(* Logix 5000 AddOnInstructionDefinition export NORD_VFDcontrol_PRO_Inst100_101; software revision 24.02 *)

TYPE FI_Data_IN :
STRUCT
   ConnectionFaulted : BOOL;
   RunMode : BOOL;
   Data : INT[6];   // Actual Values
END_STRUCT
END_TYPE

TYPE FI_Data_OUT :
STRUCT
   Data : INT[6];   // Control Data
END_STRUCT
END_TYPE

ADD_ON_INSTRUCTION NORD_VFDcontrol_PRO_Inst100_101   (* revision 1.1, vendor NORD Drivesystems, ExecutePrescan *)
// Control Block for NORD SK 5xxP VFD
// Revision note:
// Rev 1.1
// Better Ready Start Condition Logic
// Added Inhibited Output
// Added Fault Active Output
// Rev 1.0
// Connection to SK550P
// Instances: Output 100/Input 101
// For VFD Series:
//    - PRO (SK 500P Series)
// Allows for control of up to four (8) VFDs.
//    - FI_Control/Status may require Data Type change
VAR_IN_OUT
   FI_Status : _0342:XU5_EIP_DE5BFA94:I:0; {required}   // Input Data Map of VFD
   FI_Control : _0342:XU5_EIP_E8E6FFA2:O:0; {required}   // Output Data Map of VFD
END_VAR
VAR_INPUT
   Max_VFD_Number : SINT := 1;   // Maximum Number of VFDs on this specific node (1-8 for Instance 100/101)
   VFD_Number : SINT := 1; {visible}   // Number of VFD to control (1...Max_VFD_Number) for Instance 102/103)
   EnableFwd : BOOL; {visible}   // HIGH = Enable CW
   EnableRev : BOOL; {visible}   // HIGH = Enable CCW
   DisableVoltage : BOOL := 1; {visible}   // LOW = Output Voltage Disabled
   QuickStop : BOOL := 1; {visible}   // LOW = Emergency Stop Active
   FaultAckn : BOOL; {visible}   // Error / Fault Acknowledgement on Rising Edge
   ParameterSet : SINT := 1; {visible}   // Parameter Set 1-4, If less than 1 or higher than 4, Set 1 as active
        .1   // Parameter Set 1-4, If less than 1 or higher than 4, Set 1 as active
   Activate32BitSetpoint : BOOL; {visible}   // Use 32Bit Setpoint
   ControlWordBit8_P480_11 : BOOL; {visible}   // P480_11 - Function
   ControlWordBit9_P480_12 : BOOL; {visible}   // P480_12 - Function
   ControlWord : ALIAS FOR Control_Word; {access None, visible}
   Setpoint1 : INT; {visible}   // Setpoint 1 Function set in P546[1]
   Setpoint2 : INT; {visible}   // Setpoint 2 Function set in P546[2]
   Setpoint3 : INT; {visible}   // Setpoint 3 Function set in P546[3]
   Setpoint2_3_32 : DINT; {visible}   // 32 Bit Setpoint 2
   Setpoint4 : INT; {visible}   // Setpoint 4 Function set in P546[4]
   Setpoint5 : INT; {visible}   // Setpoint 5 Function set in P546[5]
END_VAR
VAR_OUTPUT
   StatusWord : INT; {access Read Only, visible}   // Status Word
        .0   // Ready to Start
        .1   // Ready for Operation
        .2   // Operation Enabled
        .3   // Fault
        .4   // Voltage Enabled
        .5   // No Emergency Stop
        .6   // Starting Disabled
        .7   // Warning Active
        .8   // Setpoint Reached
        .9   // Bus Controller Active
        .10   // Function P481[9]
        .11   // Rotation Right Active
        .12   // Rotation Left Active
        .13   // Function P481[10]
        .14   // Parameter Set Bit 0
        .15   // Parameter Set Bit 1
   ActiveParameterSet : SINT; {access Read Only, visible}   // Displays active parameter set
   CommunicationOK : BOOL; {access Read Only, visible}   // Communication is OK
   ReadyToStart : BOOL; {access Read Only, visible}   // Drive Ready to Start
   VFD_Enabled : BOOL; {access Read Only, visible}   // VFD is Enabled
   Inhibited : BOOL; {access Read Only, visible}   // VFD is Inhibited
   Warning : BOOL; {access Read Only, visible}   // Drive has a Warning
   Faulted : BOOL; {access Read Only, visible}   // Drive Faulted
   FaultActive : BOOL; {access Read Only, visible}   // Fault Conditions are Currently Active
   StatusWordBit10_P481_9 : BOOL; {access Read Only, visible}   // P481_09 - Function
   StatusWordBit13_P481_10 : BOOL; {access Read Only, visible}   // P481_10 - Function
   ActualValue1 : INT; {access Read Only, visible}   // Actual Value 1 Function set in P543[1]
   ActualValue2 : INT; {access Read Only, visible}   // Actual Value 2 Function set in P543[2]
   ActualValue3 : INT; {access Read Only, visible}   // Actual Value 3 Function set in P543[3]
   ActualValue2_3_32 : DINT; {access Read Only, visible}   // 32 Bit Actual Value 2
   ActualValue4 : INT; {access Read Only, visible}   // Actual Value 4 Function set in P543[4]
   ActualValue5 : INT; {access Read Only, visible}   // Actual Value 5 Function set in P543[5]
END_VAR
VAR
   Index : INT; {access None}   // Index of process data based on VFD address
   Control_Word : INT; {access None}   // Control Word
        .0   // Enable Operation
        .1   // Disable Voltage (Low level disables the output voltage of the drive and stops the VFD)
        .2   // Emergency Stop (Low level activates QuickStop mode and stops the VFD)
        .3   // Ready for Operation
        .4   // Enable Pulses
        .5   // Enable Ramp
        .6   // Enable Setpoint
        .7   // Error Acknowledge
        .8   // Function P480[11]
        .9   // Function P480[12]
        .10   // Control Data Valid
        .11   // Rotation Direction Clockwise
        .12   // Rotation Direction Counter-Clockwise
        .13   // Reserved
        .14   // Parameter Set Bit 0
        .15   // Parameter Set Bit 1
   Control : FI_Data_OUT; {access None}
   Status : FI_Data_IN; {access None}
   LowWordOf32BitSetpoint : DINT; {access None}
   Temporary_Variable_32BitSepoint : DINT; {access None}
   HighWordOf32BitSetpoint : DINT; {access None}
   FI_Control_Size : INT; {access None}   // Size of Output Process Data
   FI_Status_Size : INT; {access None}   // Size of Input Process Data
END_VAR

ROUTINE Logic   (* ladder *)
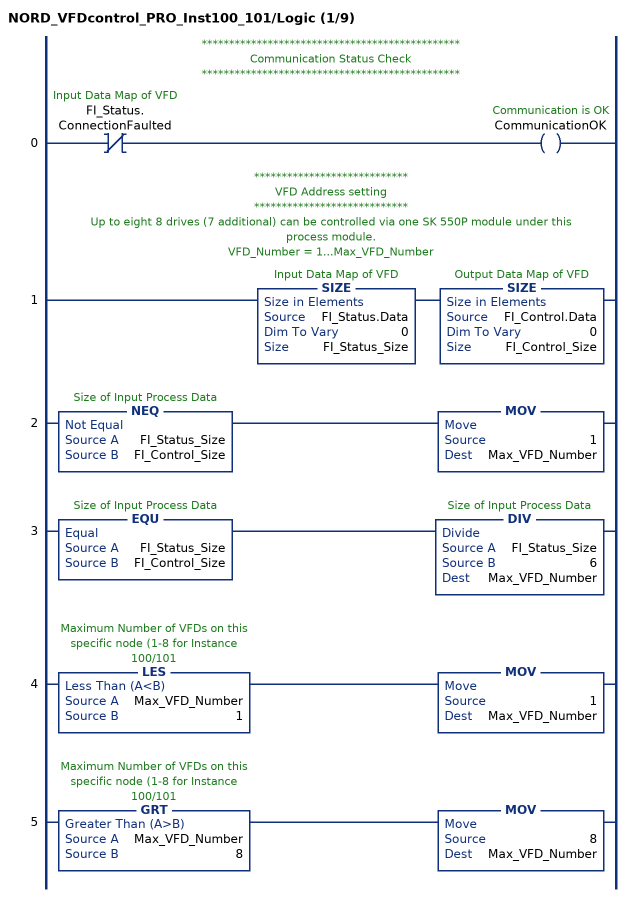
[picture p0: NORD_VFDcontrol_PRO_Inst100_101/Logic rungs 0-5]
   // ***********************************************
   // Communication Status Check
   // ***********************************************
   0: XIO(FI_Status.ConnectionFaulted)OTE(CommunicationOK);
   // ****************************
   // VFD Address setting
   // ****************************
   // Up to eight 8 drives (7 additional) can be controlled via one SK 550P module under this process module.
   // VFD_Number = 1...Max_VFD_Number
   1: SIZE(FI_Status.Data,0,FI_Status_Size)SIZE(FI_Control.Data,0,FI_Control_Size);
   2: NEQ(FI_Status_Size,FI_Control_Size)MOV(1,Max_VFD_Number);
   3: EQU(FI_Status_Size,FI_Control_Size)DIV(FI_Status_Size,6,Max_VFD_Number);
   4: LES(Max_VFD_Number,1)MOV(1,Max_VFD_Number);
   5: GRT(Max_VFD_Number,8)MOV(8,Max_VFD_Number);
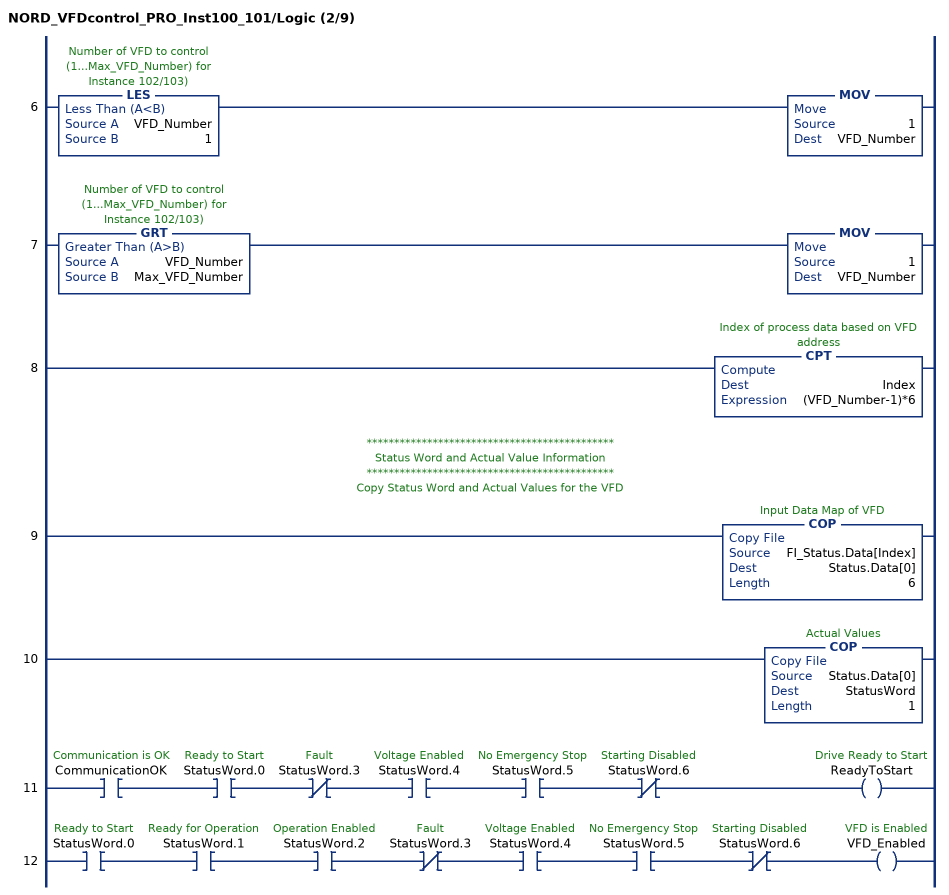
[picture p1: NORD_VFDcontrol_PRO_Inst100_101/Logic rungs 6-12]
   6: LES(VFD_Number,1)MOV(1,VFD_Number);
   7: GRT(VFD_Number,Max_VFD_Number)MOV(1,VFD_Number);
   8: CPT(Index,(VFD_Number-1)*6);
   // *********************************************
   // Status Word and Actual Value Information
   // *********************************************
   // Copy Status Word and Actual Values for the VFD
   9: COP(FI_Status.Data[Index],Status.Data[0],6);
   10: COP(Status.Data[0],StatusWord,1);
   11: XIC(CommunicationOK)XIC(StatusWord.0)XIO(StatusWord.3)XIC(StatusWord.4)XIC(StatusWord.5)XIO(StatusWord.6)OTE(ReadyToStart);
   12: XIC(StatusWord.0)XIC(StatusWord.1)XIC(StatusWord.2)XIO(StatusWord.3)XIC(StatusWord.4)XIC(StatusWord.5)XIO(StatusWord.6)OTE(VFD_Enabled);
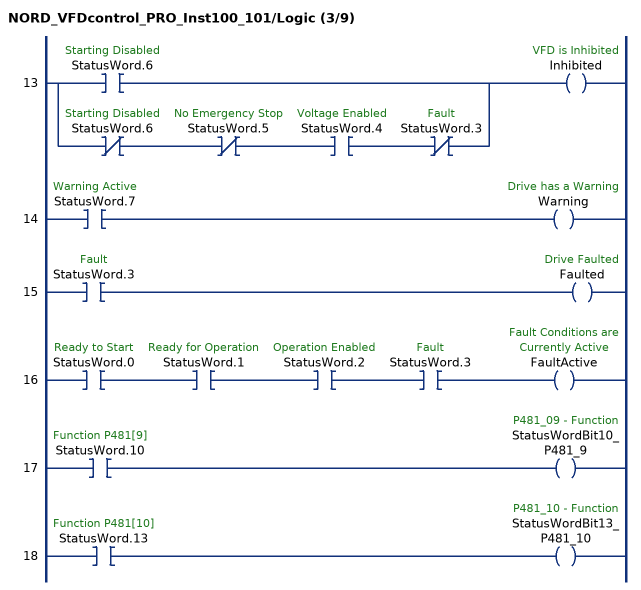
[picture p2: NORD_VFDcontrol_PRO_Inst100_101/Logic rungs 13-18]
   13: [XIC(StatusWord.6) ,XIO(StatusWord.6) XIO(StatusWord.5) XIC(StatusWord.4) XIO(StatusWord.3) ]OTE(Inhibited);
   14: XIC(StatusWord.7)OTE(Warning);
   15: XIC(StatusWord.3)OTE(Faulted);
   16: XIC(StatusWord.0)XIC(StatusWord.1)XIC(StatusWord.2)XIC(StatusWord.3)OTE(FaultActive);
   17: XIC(StatusWord.10)OTE(StatusWordBit10_P481_9);
   18: XIC(StatusWord.13)OTE(StatusWordBit13_P481_10);
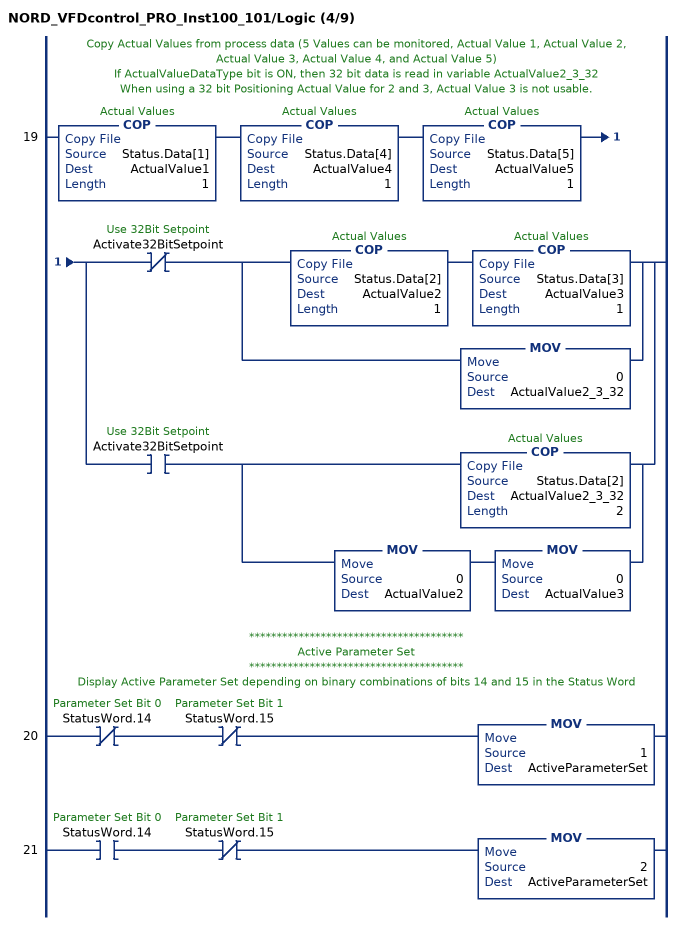
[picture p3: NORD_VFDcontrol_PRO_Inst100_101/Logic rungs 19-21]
   // Copy Actual Values from process data (5 Values can be monitored, Actual Value 1, Actual Value 2, Actual Value 3, Actual Value 4, and Actual Value 5)
   // If ActualValueDataType bit is ON, then 32 bit data is read in variable ActualValue2_3_32
   // When using a 32 bit Positioning Actual Value for 2 and 3, Actual Value 3 is not usable.
   19: COP(Status.Data[1],ActualValue1,1)COP(Status.Data[4],ActualValue4,1)COP(Status.Data[5],ActualValue5,1)[XIO(Activate32BitSetpoint) [COP(Status.Data[2],ActualValue2,1) COP(Status.Data[3],ActualValue3,1) ,MOV(0,ActualValue2_3_32) ] ,XIC(Activate32BitSetpoint) [COP(Status.Data[2],ActualValue2_3_32,2) ,MOV(0,ActualValue2) MOV(0,ActualValue3) ] ];
   // ***************************************
   // Active Parameter Set
   // ***************************************
   // Display Active Parameter Set depending on binary combinations of bits 14 and 15 in the Status Word
   20: XIO(StatusWord.14)XIO(StatusWord.15)MOV(1,ActiveParameterSet);
   21: XIC(StatusWord.14)XIO(StatusWord.15)MOV(2,ActiveParameterSet);
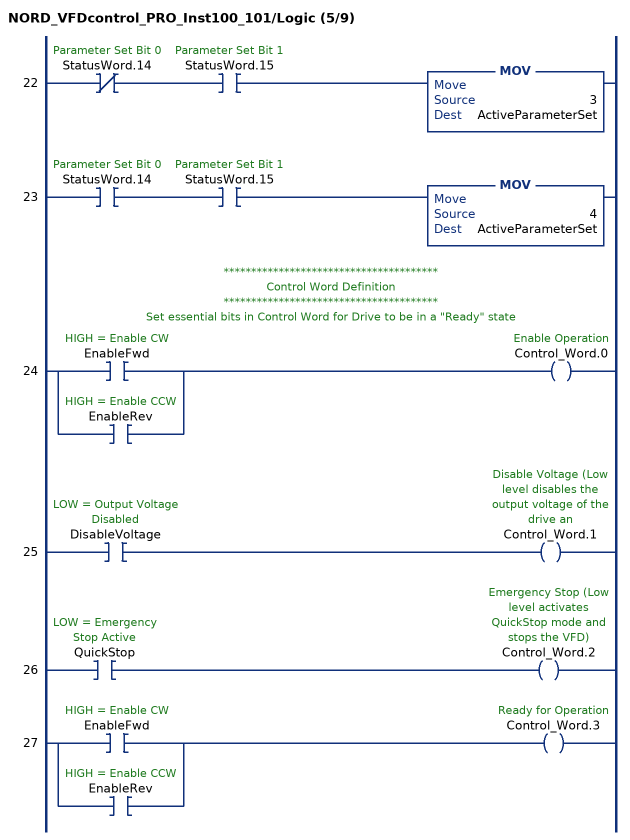
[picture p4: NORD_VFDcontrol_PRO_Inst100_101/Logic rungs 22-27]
   22: XIO(StatusWord.14)XIC(StatusWord.15)MOV(3,ActiveParameterSet);
   23: XIC(StatusWord.14)XIC(StatusWord.15)MOV(4,ActiveParameterSet);
   // ***************************************
   // Control Word Definition
   // ***************************************
   // Set essential bits in Control Word for Drive to be in a "Ready" state
   24: [XIC(EnableFwd) ,XIC(EnableRev) ]OTE(Control_Word.0);
   25: XIC(DisableVoltage)OTE(Control_Word.1);
   26: XIC(QuickStop)OTE(Control_Word.2);
   27: [XIC(EnableFwd) ,XIC(EnableRev) ]OTE(Control_Word.3);
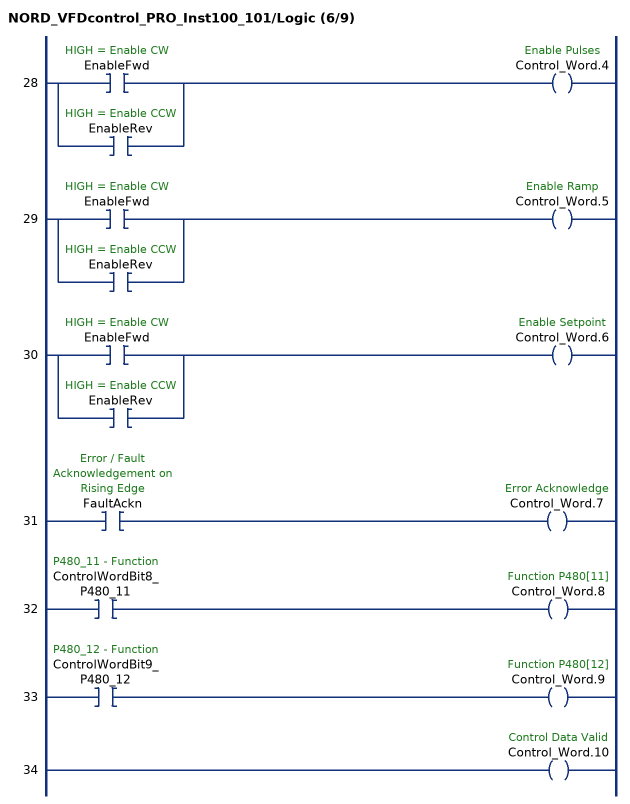
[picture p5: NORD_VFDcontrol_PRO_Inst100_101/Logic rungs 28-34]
   28: [XIC(EnableFwd) ,XIC(EnableRev) ]OTE(Control_Word.4);
   29: [XIC(EnableFwd) ,XIC(EnableRev) ]OTE(Control_Word.5);
   30: [XIC(EnableFwd) ,XIC(EnableRev) ]OTE(Control_Word.6);
   31: XIC(FaultAckn)OTE(Control_Word.7);
   32: XIC(ControlWordBit8_P480_11)OTE(Control_Word.8);
   33: XIC(ControlWordBit9_P480_12)OTE(Control_Word.9);
   34: OTE(Control_Word.10);
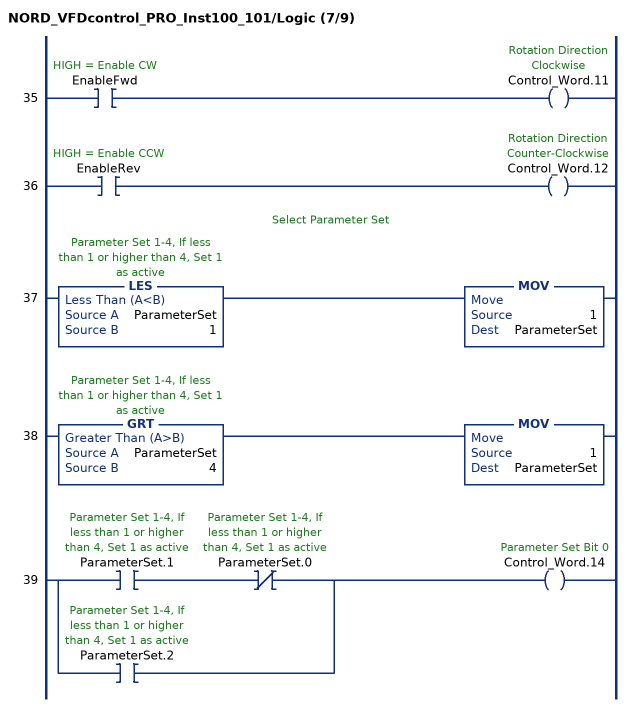
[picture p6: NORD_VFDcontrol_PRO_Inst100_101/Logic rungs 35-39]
   35: XIC(EnableFwd)OTE(Control_Word.11);
   36: XIC(EnableRev)OTE(Control_Word.12);
   // Select Parameter Set
   37: LES(ParameterSet,1)MOV(1,ParameterSet);
   38: GRT(ParameterSet,4)MOV(1,ParameterSet);
   39: [XIC(ParameterSet.1) XIO(ParameterSet.0) ,XIC(ParameterSet.2) ]OTE(Control_Word.14);
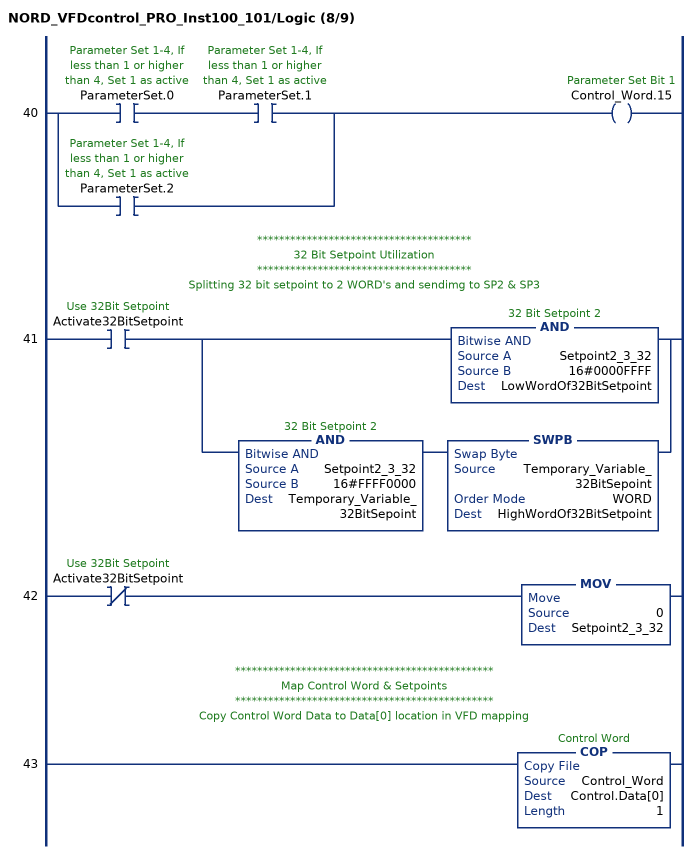
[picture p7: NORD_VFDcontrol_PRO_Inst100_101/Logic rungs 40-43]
   40: [XIC(ParameterSet.0) XIC(ParameterSet.1) ,XIC(ParameterSet.2) ]OTE(Control_Word.15);
   // ***************************************
   // 32 Bit Setpoint Utilization
   // ***************************************
   // Splitting 32 bit setpoint to 2 WORD's and sendimg to SP2 & SP3
   41: XIC(Activate32BitSetpoint)[AND(Setpoint2_3_32,16#0000FFFF,LowWordOf32BitSetpoint) ,AND(Setpoint2_3_32,16#FFFF0000,Temporary_Variable_32BitSepoint) SWPB(Temporary_Variable_32BitSepoint,WORD,HighWordOf32BitSetpoint) ];
   42: XIO(Activate32BitSetpoint)MOV(0,Setpoint2_3_32);
   // ***********************************************
   // Map Control Word & Setpoints
   // ***********************************************
   // Copy Control Word Data to Data[0] location in VFD mapping
   43: COP(Control_Word,Control.Data[0],1);
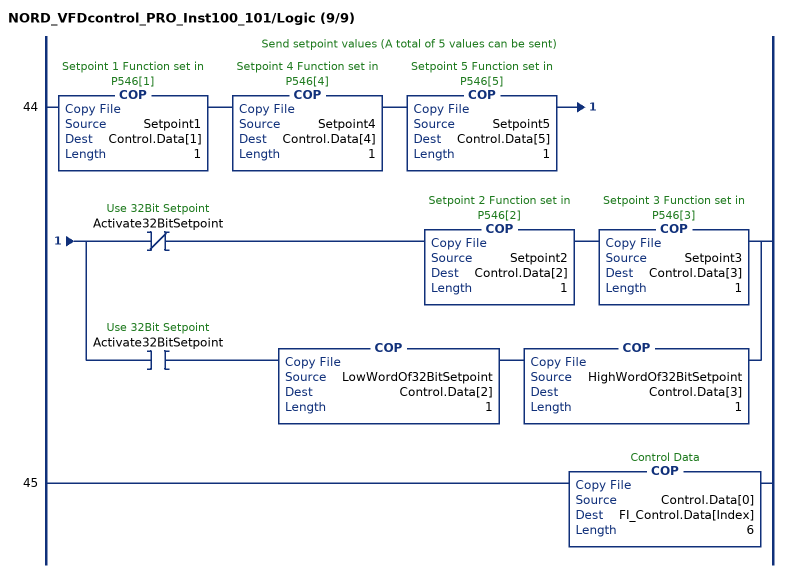
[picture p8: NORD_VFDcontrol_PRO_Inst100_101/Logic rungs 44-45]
   // Send setpoint values (A total of 5 values can be sent)
   44: COP(Setpoint1,Control.Data[1],1)COP(Setpoint4,Control.Data[4],1)COP(Setpoint5,Control.Data[5],1)[XIO(Activate32BitSetpoint) COP(Setpoint2,Control.Data[2],1) COP(Setpoint3,Control.Data[3],1) ,XIC(Activate32BitSetpoint) COP(LowWordOf32BitSetpoint,Control.Data[2],1) COP(HighWordOf32BitSetpoint,Control.Data[3],1) ];
   45: COP(Control.Data[0],FI_Control.Data[Index],6);
END_ROUTINE

ROUTINE Prescan   (* ladder *)
// Executed prior to first scan of AOI
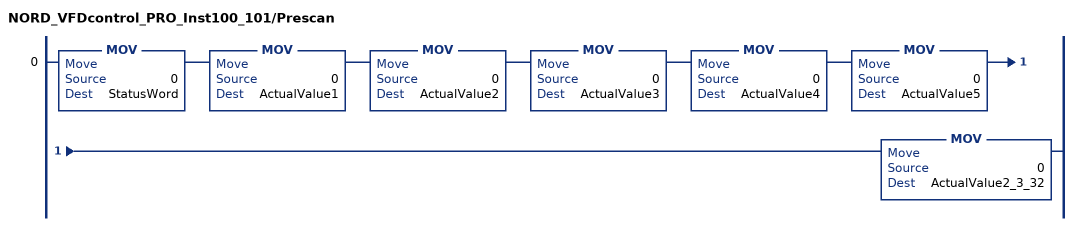
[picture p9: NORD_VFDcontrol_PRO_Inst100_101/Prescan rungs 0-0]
   0: MOV(0,StatusWord)MOV(0,ActualValue1)MOV(0,ActualValue2)MOV(0,ActualValue3)MOV(0,ActualValue4)MOV(0,ActualValue5)MOV(0,ActualValue2_3_32);
END_ROUTINE
END_ADD_ON_INSTRUCTION
